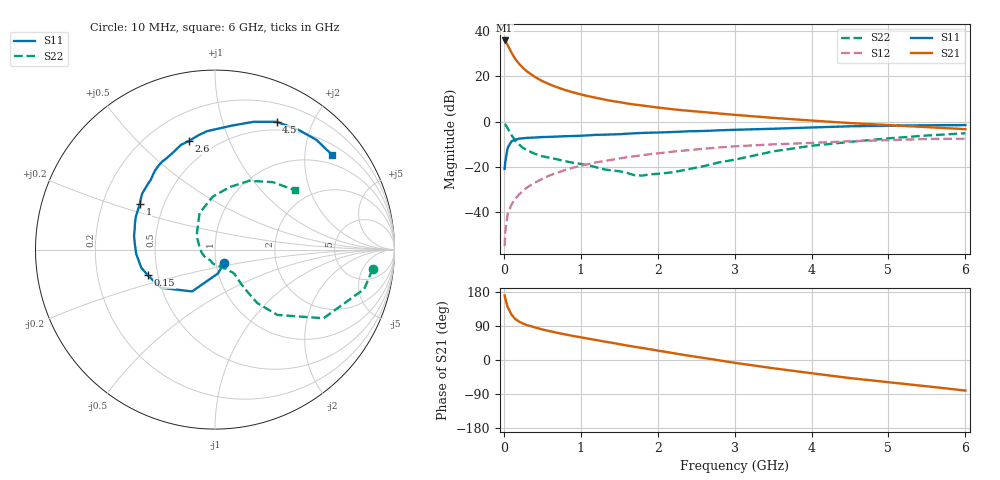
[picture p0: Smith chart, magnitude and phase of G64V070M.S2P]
! SIEMENS Small Signal Semiconductors
! BFG193
! Si NPN RF Bipolar Junction Transistor in SOT223
! VCE = 4 V  IC = 70 mA
! Common Emitter S-Parameters:  August  1996
# GHz  S  MA  R  50
!  f  S11  S21  S12  S22
! GHz  MAG  ANG  MAG  ANG  MAG  ANG  MAG  ANG
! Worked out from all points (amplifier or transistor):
!   36 points, 10 MHz to 6 GHz, reference 50 ohm
!   highest |S21| = 35.8 dB at 10 MHz (marker M1)
!   |S21| within 3 dB of that: start of sweep to 63.69 MHz
!   unconditionally stable (mu >= 1): 346.8 MHz to 2.325 GHz
!   at 250 MHz: K = 0.97, MSG = 27.1 dB, |S12| = -30.5 dB
!   at 1.4 GHz: K = 1.05, MAG = 11.6 dB, |S12| = -16.8 dB
!   at 6 GHz: K = 0.91, MSG = 2.1 dB, |S12| = -7.5 dB
!   S11 on the Smith chart (normalised r, x): 10 MHz: 1.09, -0.17; 150 MHz: 0.44, -0.15; 1 GHz: 0.37, +0.24; 2.6 GHz: 0.37, +0.72; 4.5 GHz: 0.40, +1.52; 6 GHz: 0.75, +2.65
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0.01  0.0908 -55.8  61.66 170.2  0.0018 81.3  0.8845 -7.1
0.02  0.1342 -83.2  59.14 161.6  0.0039 73.5  0.8599 -14.8
0.05  0.2658 -118.7  48.47 139.6  0.0091 72.1  0.7157 -32.3
0.1  0.3696 -144.9  33.07 119.7  0.015 69.2  0.5035 -46.3
0.15  0.4003 -159.0  23.94 107.8  0.0199 68.8  0.3793 -51.7
0.2  0.4231 -166.2  18.74 101.2  0.0251 70.8  0.3121 -52.3
0.25  0.4299 -172.0  15.24 96.1  0.0298 70.7  0.2634 -52.7
0.3  0.4396 -176.8  12.86 92.1  0.0353 71.4  0.2364 -52.7
0.4  0.4471 176.4  9.772 86.3  0.0449 71.6  0.1962 -51.9
0.5  0.4577 170.3  7.845 80.6  0.0549 70.2  0.1731 -51.4
0.6  0.4618 165.7  6.593 76.0  0.0657 69.3  0.1597 -52.6
0.7  0.4698 161.5  5.67 71.5  0.0754 67.5  0.147 -55.1
0.8  0.4781 157.2  4.957 67.4  0.0861 65.4  0.1343 -57.1
1  0.4896 148.9  3.993 59.9  0.1062 61.9  0.1171 -63.2
1.1  0.4995 146.1  3.635 56.3  0.1159 60.1  0.1087 -69.1
1.6  0.5426 129.4  2.518 38.2  0.1644 48.9  0.0744 -102.8
2.2  0.5915 112.8  1.872 18.2  0.2186 35.2  0.0767 -168.2
2.6  0.6229 103.3  1.624 5.4  0.2523 26.3  0.1047 154.1
3.5  0.6974 82.2  1.213 -21.7  0.3159 3.6  0.2209 112.9
4.5  0.7902 64.3  0.931 -47.7  0.3709 -16.5  0.3586 76.6
5.5  0.8325 47.2  0.758 -69.4  0.416 -40.1  0.4952 49.4
6  0.8393 38.8  0.683 -80.7  0.4207 -53.6  0.5554 36.4
